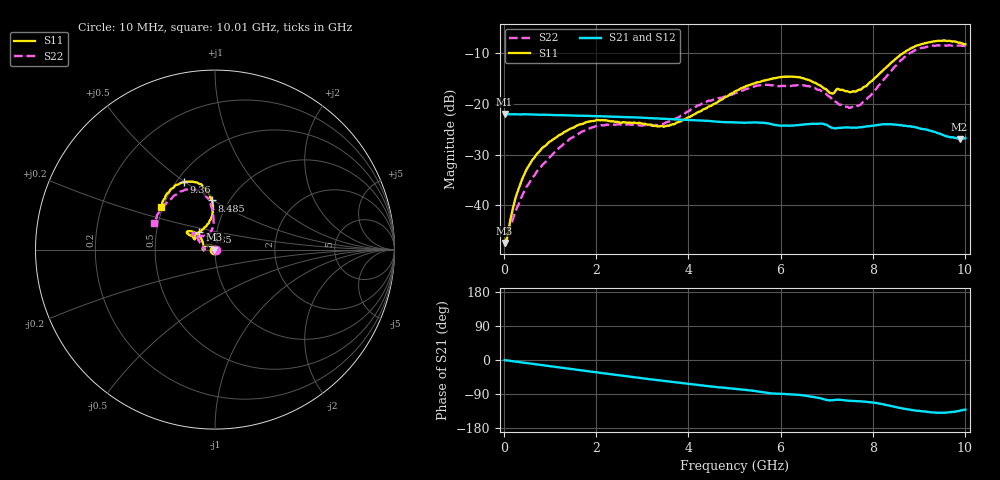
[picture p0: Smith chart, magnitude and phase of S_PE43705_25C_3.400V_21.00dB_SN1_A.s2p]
! Device ID: PE43705
! Serial: 1
! Insertion: A
! Impedance: 50 ohm
! Temp: 25C
! VDD: 3.400V
! Attenuation Step: 21.00dB
#  Hz  S  RI  R  50
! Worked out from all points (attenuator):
!   401 points, 10 MHz to 10.01 GHz, reference 50 ohm
!   highest |S21| = -22.03 dB at 10 MHz (marker M1); lowest = -27.0 dB at 9.885 GHz (marker M2)
!   lowest |S11| = -47.4 dB at 10 MHz (marker M3), VSWR 1.01, Z = 49.6 + j0.047 ohm
!   |S11| at or under -10 dB: start of sweep to 8.665 GHz
!   |S22| runs from -48.0 to -8.5 dB; largest |S21 - S12| = 0.00084
!   S11 on the Smith chart (normalised r, x): 10 MHz: 0.99, +0.00; 7.435 GHz: 0.82, +0.16; 8.485 GHz: 0.83, +0.49; 9.36 GHz: 0.55, +0.50; 10.01 GHz: 0.49, +0.27
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1e7  -0.00424 0.000474  0.0792 -0.000259  0.0792 -0.00032  0.00394 0.0004
6e7  -0.004 0.00259  0.079 -0.00156  0.079 -0.00154  0.00421 0.00192
2.85e8  -0.00596 0.012  0.0784 -0.00667  0.0783 -0.0066  0.00212 0.00933
5.85e8  -0.0142 0.0228  0.0771 -0.0134  0.0772 -0.0133  -0.00559 0.0171
1.01e9  -0.033 0.0274  0.0743 -0.0225  0.0743 -0.0225  -0.0239 0.0187
1.685e9  -0.0607 0.0172  0.0676 -0.0352  0.0676 -0.0352  -0.0524 0.00859
2.185e9  -0.0686 0.00313  0.0611 -0.0435  0.0612 -0.0435  -0.0613 -0.00152
3.36e9  -0.0596 0.00398  0.0423 -0.0576  0.0424 -0.0575  -0.0614 0.00836
3.86e9  -0.0628 0.0269  0.0337 -0.0608  0.0339 -0.0608  -0.0726 0.0265
5.01e9  -0.0995 0.0871  0.0157 -0.0636  0.0157 -0.0635  -0.1042 0.0729
5.535e9  -0.1292 0.1002  0.00743 -0.0647  0.00752 -0.0646  -0.122 0.0892
6.01e9  -0.1523 0.1018  0.000853 -0.0607  0.0011 -0.0609  -0.1201 0.089
6.685e9  -0.1432 0.0819  -0.00773 -0.0631  -0.00783 -0.063  -0.1196 0.0809
7.085e9  -0.1097 0.0649  -0.0165 -0.0565  -0.0167 -0.0564  -0.084 0.079
7.435e9  -0.091 0.0968  -0.0171 -0.0557  -0.0167 -0.0559  -0.0484 0.0804
7.785e9  -0.0453 0.1366  -0.0199 -0.0554  -0.0197 -0.0556  -0.0229 0.1012
8.36e9  -0.0111 0.2441  -0.0318 -0.0542  -0.0316 -0.0544  -0.0117 0.2018
8.485e9  -0.017 0.2741  -0.0347 -0.052  -0.0346 -0.0519  -0.0193 0.2336
8.885e9  -0.0696 0.3536  -0.0403 -0.0436  -0.0397 -0.0438  -0.0771 0.3207
9.36e9  -0.1717 0.3757  -0.0397 -0.0345  -0.0395 -0.0344  -0.181 0.3263
9.885e9  -0.2854 0.2804  -0.031 -0.0324  -0.0314 -0.0324  -0.3166 0.2017
1.001e10  -0.3021 0.2385  -0.0303 -0.0349  -0.0302 -0.0349  -0.3411 0.1503
